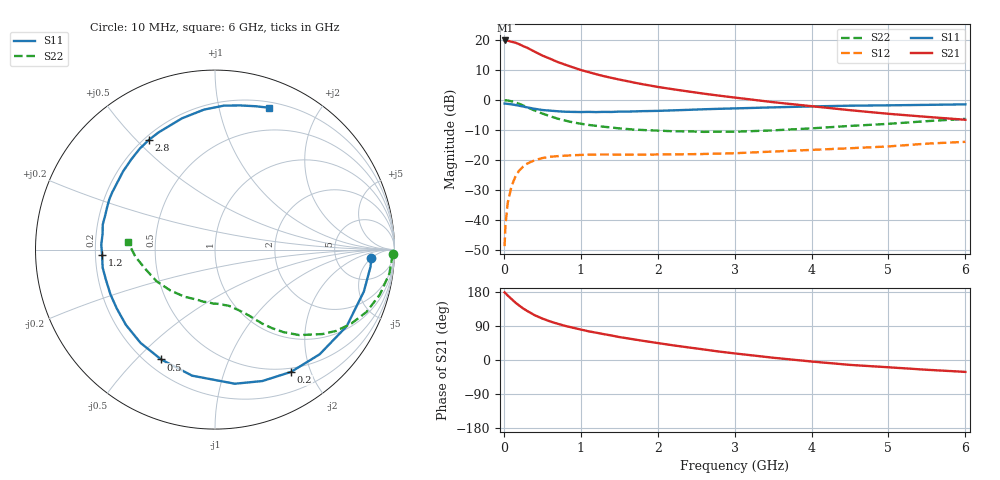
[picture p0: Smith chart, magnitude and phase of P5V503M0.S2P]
! SIEMENS Small Signal Semiconductors
! BFP183
! Si NPN RF Bipolar Junction Transistor in SOT143
! VCE = 0.5 V  IC = 3 mA
! Common Emitter S-Parameters:  March  1996
# GHz  S  MA  R  50
!  f  S11  S21  S12  S22
! GHz  MAG  ANG  MAG  ANG  MAG  ANG  MAG  ANG
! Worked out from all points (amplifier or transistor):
!   36 points, 10 MHz to 6 GHz, reference 50 ohm
!   highest |S21| = 19.8 dB at 20 MHz (marker M1)
!   |S21| within 3 dB of that: start of sweep to 346.1 MHz
!   unconditionally stable (mu >= 1): 1.67 GHz to end of sweep
!   at 250 MHz: K = 0.17, MSG = 20.1 dB, |S12| = -22.2 dB
!   at 1.4 GHz: K = 0.86, MSG = 12.8 dB, |S12| = -18.1 dB
!   at 6 GHz: K = 1.20, MAG = 1.0 dB, |S12| = -13.9 dB
!   S11 on the Smith chart (normalised r, x): 10 MHz: 13, -5; 200 MHz: 0.45, -1.71; 500 MHz: 0.26, -0.59; 1.2 GHz: 0.23, -0.02; 2.8 GHz: 0.22, +0.54; 6 GHz: 0.26, +1.42
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0.01  0.8722 -3.1  9.685 178.4  0.0037 84.6  0.9921 -1.5
0.02  0.8718 -6.3  9.786 176.7  0.008 85.6  0.9869 -3.1
0.05  0.8616 -15.7  9.704 170.2  0.0194 83.0  0.9806 -7.9
0.1  0.8489 -30.2  9.311 160.9  0.0368 73.6  0.952 -15.3
0.15  0.8248 -45.0  8.997 151.6  0.0532 65.2  0.9126 -22.4
0.2  0.8024 -58.1  8.474 143.6  0.0671 58.8  0.8647 -28.4
0.25  0.7784 -70.2  7.885 136.2  0.0778 52.5  0.8138 -33.8
0.3  0.7554 -81.6  7.43 129.9  0.0869 47.7  0.761 -38.2
0.4  0.7139 -100.3  6.383 118.3  0.0995 39.3  0.6689 -45.4
0.5  0.6816 -116.1  5.494 109.4  0.1082 33.0  0.5964 -50.4
0.6  0.665 -128.6  4.868 101.9  0.1136 28.5  0.5379 -54.2
0.7  0.6499 -139.8  4.283 95.6  0.1165 24.7  0.4897 -57.4
0.8  0.6381 -149.0  3.861 89.9  0.1186 21.8  0.4533 -59.7
1.1  0.634 -170.9  2.914 75.8  0.1232 16.0  0.3853 -65.5
1.2  0.6297 -177.2  2.686 72.1  0.1237 14.1  0.3716 -67.4
1.7  0.6459 158.5  1.94 54.1  0.1228 11.3  0.321 -76.7
2.2  0.6725 139.6  1.509 38.7  0.1245 10.5  0.3022 -87.4
2.8  0.7135 121.2  1.181 22.2  0.1285 11.3  0.2978 -102.5
3.5  0.7542 104.1  0.92 6.0  0.1388 12.4  0.3124 -122.7
4.5  0.8039 86.4  0.677 -12.9  0.1575 11.5  0.3703 -151.5
5.5  0.8298 74.3  0.524 -25.8  0.1879 9.2  0.4448 -174.8
6  0.8463 69.0  0.469 -31.4  0.2015 6.0  0.4853 175.2
